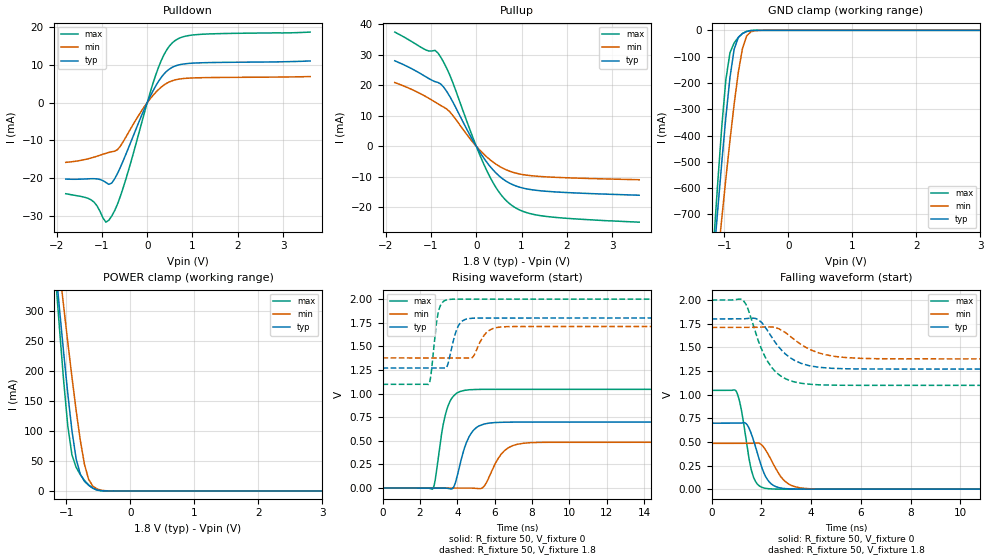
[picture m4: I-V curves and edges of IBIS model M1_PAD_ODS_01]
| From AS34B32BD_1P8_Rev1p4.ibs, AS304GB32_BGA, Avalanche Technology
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[Model] M1_PAD_ODS_01
Model_type I/O
Enable   Active-High
Vinl  =  0.63
Vinh  =  1.17
Vmeas =  0.9
Cref  =  30e-12
| Capacitance  typ   min   max
C_comp   6.492186e-12   6.071794e-12   6.967131e-12
| Variables   typ   min   max
[GND Clamp Reference]   0   0   0
[POWER Clamp Reference]   1.8   1.71   2
[Pulldown Reference]   0   0   0
[Pullup Reference]   1.8   1.71   2
[Temperature Range]   25   125   -40
[Voltage Range]   1.8   1.71   2
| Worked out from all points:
|   slope of the pulldown table from 0 to 0.27 V, typ, clamps not added: 44.9 ohm
|   slope of the pullup table from 0 to 0.27 V, typ, clamps not added: 45.3 ohm
|   GND clamp passes 1 mA (typ) near -0.58 V on its own axis
|   POWER clamp passes 1 mA (typ) near -0.48 V on its own axis
|   falling waveform, R_fixture 50, V_fixture 0: 20-80 % time 528ps typ, 663ps min, 395ps max; typ from 0.698 V to 0 V
|   falling waveform, R_fixture 50, V_fixture 1.8: 20-80 % time 1.04ns typ, 1.25ns min, 873ps max; typ from 1.8 V to 1.27 V
|   rising waveform, R_fixture 50, V_fixture 0: 20-80 % time 667ps typ, 829ps min, 541ps max; typ from 0 V to 0.698 V
|   rising waveform, R_fixture 50, V_fixture 1.8: 20-80 % time 426ps typ, 560ps min, 305ps max; typ from 1.27 V to 1.8 V
[GND Clamp]
| Voltage   I(typ)   I(min)   I(max)
-1.8V     -2.882A    -2.682A    -3.302A
-1.173V   -889.3mA   -1.041A    -830.7mA
-1.108V   -695.2mA   -879.1mA   -594mA
-1.043V   -507.9mA   -720.4mA   -373.2mA
-977.6mV  -332.2mA   -566.2mA   -188.7mA
-912.4mV  -178.9mA   -418.3mA   -84.9mA
-847.2mV  -71.94mA   -280.4mA   -47.66mA
-782.1mV  -27.06mA   -159.4mA   -26.61mA
-716.9mV  -11.75mA   -68.54mA   -12.18mA
-651.7mV  -4.473mA   -21mA      -3.801mA
-456.2mV  -15.91uA   -297.6uA   -1.681uA
3.6V      0A         0A         0A
[POWER Clamp]
| Voltage   I(typ)   I(min)   I(max)
-1.8V     1.148A     1.073A     1.318A
-1.173V   379.5mA    433.8mA    364.1mA
-1.108V   304.4mA    370.6mA    271.9mA
-1.043V   231.6mA    308.7mA    184.6mA
-977.6mV  162.5mA    248.2mA    108.6mA
-912.4mV  100.5mA    189.8mA    60.25mA
-847.2mV  53.5mA     134.6mA    39.41mA
-716.9mV  16.06mA    44.37mA    17.57mA
-651.7mV  9.361mA    19.28mA    9.931mA
-586.6mV  4.721mA    8.013mA    4.451mA
-325.9mV  4.613uA    79.39uA    440.6nA
3.6V      0A         0A         0A
[Pulldown]
| Voltage   I(typ)   I(min)   I(max)
-1.8V     -20.26mA   -15.83mA   -24.15mA
-1.238V   -20.17mA   -14.67mA   -25.78mA
-912.4mV  -21.17mA   -13.42mA   -31.69mA
-847.2mV  -21.66mA   -13.2mA    -31.16mA
-716.9mV  -20.14mA   -12.86mA   -28.56mA
-521.4mV  -15.14mA   -10.15mA   -22.2mA
-65.17mV  -1.742mA   -1.091mA   -2.802mA
248.3mV   5.63mA     3.46mA     9.353mA
434.5mV   8.383mA    5.171mA    14.07mA
620.7mV   9.735mA    6.051mA    16.51mA
1.179V    10.57mA    6.614mA    18.12mA
3.6V      11.06mA    6.923mA    18.71mA
[Pullup]
| Voltage   I(typ)   I(min)   I(max)
-1.8V     28.03mA    20.89mA    37.45mA
-1.108V   22.74mA    16.24mA    31.55mA
-912.4mV  21.2mA     14.52mA    31.47mA
-782.1mV  20.39mA    13.35mA    29.17mA
-521.4mV  14.66mA    10.17mA    21.02mA
-130.3mV  3.403mA    2.332mA    5.058mA
186.2mV   -4.285mA   -2.877mA   -6.521mA
496.6mV   -9.629mA   -6.461mA   -14.9mA
744.8mV   -12.18mA   -8.22mA    -18.94mA
1.055V    -13.81mA   -9.36mA    -21.49mA
1.49V     -14.71mA   -9.993mA   -22.92mA
3.6V      -16.07mA   -10.99mA   -24.92mA
[Ramp]
dV/dt_r   0.418626/0.666589n  0.290552/0.828677n  0.626829/0.541304n
dV/dt_f   0.31797/1.03708n  0.199635/1.24522n  0.541445/0.873151n
R_load = 50
[Falling Waveform]
R_fixture = 50
V_fixture = 0
V_fixture_min = 0
V_fixture_max = 0
| Time   V(typ)   V(min)   V(max)
0s        697.7mV    484.3mV    1.045V
1ns       698.4mV    484.8mV    1.03V
1.217ns   699.8mV    484.9mV    809.7mV
1.616ns   570.3mV    485.1mV    184.4mV
1.833ns   387.7mV    488.2mV    55.63mV
2.108ns   169.4mV    438.8mV    12.24mV
2.397ns   56.32mV    308.2mV    2.95mV
2.892ns   7.942mV    97.61mV    356.9uV
3.789ns   578.1uV    6.943mV    163.1uV
21.88ns   -27.03nV   427.3nV    -12.25nV
[Falling Waveform]
R_fixture = 50
V_fixture = 1.8
V_fixture_min = 1.71
V_fixture_max = 2
| Time   V(typ)   V(min)   V(max)
0s        1.8V       1.71V      2V
1.28ns    1.801V     1.711V     1.994V
1.487ns   1.806V     1.711V     1.889V
1.873ns   1.794V     1.711V     1.572V
2.256ns   1.673V     1.716V     1.349V
2.747ns   1.489V     1.69V      1.203V
3.506ns   1.34V      1.546V     1.124V
4.523ns   1.284V     1.425V     1.102V
5.934ns   1.271V     1.384V     1.098V
21.88ns   1.27V      1.377V     1.098V
[Rising Waveform]
R_fixture = 50
V_fixture = 0
V_fixture_min = 0
V_fixture_max = 0
| Time   V(typ)   V(min)   V(max)
0s        5.879nV    262.4nV    4.64nV
2.701ns   -545.2uV   -376.3uV   -4.991mV
3.168ns   -639.5uV   -441.4uV   584.4mV
3.466ns   -3.118mV   -482.8uV   846.7mV
3.827ns   18.18mV    -533.1uV   978.4mV
4.362ns   408.7mV    -607.7uV   1.033V
5.181ns   658.7mV    -8.119mV   1.044V
6.513ns   696.3mV    392.9mV    1.044V
7.54ns    697.2mV    473.8mV    1.044V
21.88ns   697.7mV    484.3mV    1.045V
[Rising Waveform]
R_fixture = 50
V_fixture = 1.8
V_fixture_min = 1.71
V_fixture_max = 2
| Time   V(typ)   V(min)   V(max)
0s        1.27V      1.377V     1.098V
2.48ns    1.271V     1.377V     1.1V
2.599ns   1.271V     1.377V     1.21V
2.975ns   1.271V     1.377V     1.852V
3.474ns   1.298V     1.377V     1.994V
3.997ns   1.69V      1.377V     2V
4.597ns   1.793V     1.376V     2V
5.545ns   1.799V     1.642V     2V
6.309ns   1.799V     1.704V     2V
21.88ns   1.8V       1.71V      2V
